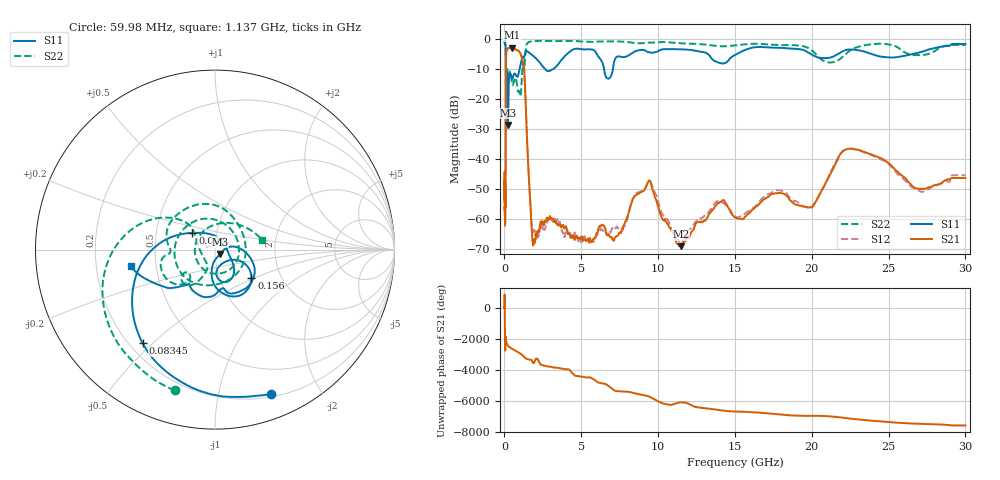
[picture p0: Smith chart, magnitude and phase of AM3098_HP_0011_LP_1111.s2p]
! Date/Time: Thu, Feb 28, 2019 8:34 AM
! Network Analyzer: Agilent Technologies E8364B Rev: A.07.50.67
! Sweep from 0.010 to 30.000 GHz, 1601 Points, Sweep Type: LOG
! Power Supply: 5.022 V, 0.002 A
# Hz S DB R 50
!freq MagS11 AngS11 MagS21 AngS21 MagS12 AngS12 MagS22 AngS22
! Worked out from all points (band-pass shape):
!   1601 points, 10 MHz to 30 GHz, reference 50 ohm
!   highest |S21| = -2.75 dB at 498 MHz (marker M1); lowest = -69.0 dB at 11.48 GHz (marker M2)
!   |S21| within 3 dB of the highest: 109.1 MHz to 1.113 GHz (1.004 GHz wide, 164 % of centre)
!   lowest |S11| = -28.5 dB at 232.8 MHz (marker M3), VSWR 1.08, Z = 52.8 - j2.63 ohm
!   |S11| at or under -10 dB: 93.02 MHz to 973.1 MHz (880.1 MHz wide, 165 % of centre); 2.667 GHz to 3.137 GHz (470 MHz wide, 16.2 % of centre); 6.491 GHz to 7.055 GHz (564.2 MHz wide, 8.33 % of centre)
!   |S22| runs from -22.3 to -0.5 dB; largest |S21 - S12| = 0.01
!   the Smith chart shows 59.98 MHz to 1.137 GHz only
!   S11 on the Smith chart (normalised r, x): 59.98 MHz: 0.23, -1.43; 83.45 MHz: 0.25, -0.47; 96 MHz: 0.76, +0.15; 156 MHz: 1.41, -0.48; 1.137 GHz: 0.36, -0.09
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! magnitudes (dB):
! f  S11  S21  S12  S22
! 10 MHz  -0.4  -47.1  -44.3  -0.6
! 38.04 MHz  -0.5  -61.8  -60.0  -1.0
! 59.98 MHz  -1.3  -51.8  -50.4  -1.8
! 73.27 MHz  -2.0  -52.0  -52.4  -2.5
! 83.45 MHz  -3.6  -36.2  -35.6  -4.0
! 96 MHz  -16.1  -12.4  -12.4  -20.0
! 144.7 MHz  -15.2  -3.6  -3.5  -13.1
! 156 MHz  -11.8  -3.5  -3.4  -11.2
! 232.8 MHz  -28.5  -2.9  -2.9  -11.9
! 308.1 MHz  -12.4  -2.9  -2.8  -11.1
! 498 MHz  -13.2  -2.8  -2.7  -14.9
! 550.5 MHz  -12.6  -2.9  -2.9  -15.1
! 1.137 GHz  -6.4  -6.2  -6.2  -11.4
! 1.308 GHz  -5.4  -12.2  -12.1  -8.9
! 1.811 GHz  -5.2  -65.5  -63.7  -0.6
! 2.084 GHz  -6.5  -64.5  -64.8  -0.5
! 7.926 GHz  -5.7  -60.2  -60.9  -0.8
! 9.443 GHz  -4.4  -47.0  -47.2  -1.1
! 11.48 GHz  -3.3  -69.0  -67.6  -1.3
! 19.7 GHz  -4.2  -55.9  -56.1  -2.7
! 22.67 GHz  -3.4  -36.4  -36.6  -3.2
! 30 GHz  -1.5  -46.2  -45.3  -1.9
